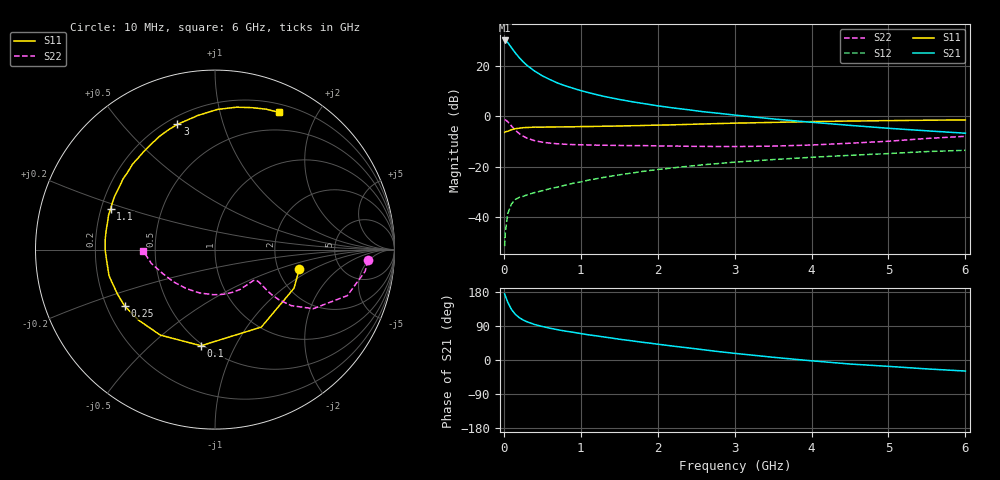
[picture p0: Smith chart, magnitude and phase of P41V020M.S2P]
! SIEMENS Small Signal Semiconductors
! BFP182
! Si NPN RF Bipolar Junction Transistor in SOT143
! VCE = 1 V  IC = 20 mA
! Common Emitter S-Parameters:  March  1996
# GHz  S  MA  R  50
!  f  S11  S21  S12  S22
! GHz  MAG  ANG  MAG  ANG  MAG  ANG  MAG  ANG
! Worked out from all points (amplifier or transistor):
!   36 points, 10 MHz to 6 GHz, reference 50 ohm
!   highest |S21| = 29.9 dB at 10 MHz (marker M1)
!   |S21| within 3 dB of that: start of sweep to 102.9 MHz
!   unconditionally stable (mu >= 1): start of sweep to 13.33 MHz; 343.8 MHz to end of sweep
!   at 250 MHz: K = 0.82, MSG = 26.6 dB, |S12| = -31.7 dB
!   at 1.4 GHz: K = 1.75, MAG = 10.4 dB, |S12| = -23.7 dB
!   at 6 GHz: K = 1.33, MAG = -0.1 dB, |S12| = -13.5 dB
!   S11 on the Smith chart (normalised r, x): 10 MHz: 2.63, -0.73; 100 MHz: 0.49, -0.74; 250 MHz: 0.27, -0.27; 1.1 GHz: 0.24, +0.18; 3 GHz: 0.24, +0.72; 6 GHz: 0.29, +1.53
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0.01  0.482 -12.8  31.39 174.3  0.0027 79.0  0.8538 -4.0
0.02  0.49 -26.1  31.28 168.8  0.0051 75.0  0.8456 -8.2
0.05  0.5029 -59.1  28.63 152.8  0.0118 68.6  0.7802 -19.2
0.1  0.5413 -98.3  22.53 133.2  0.0185 52.5  0.6391 -31.0
0.15  0.5655 -122.6  17.74 120.3  0.0226 45.2  0.5276 -36.3
0.2  0.5796 -137.3  14.37 111.8  0.0249 42.4  0.453 -38.1
0.25  0.5934 -147.9  11.92 105.6  0.026 41.0  0.4041 -38.5
0.3  0.5974 -155.5  10.13 101.0  0.0278 41.7  0.3692 -38.1
0.4  0.608 -166.0  7.797 93.7  0.031 43.5  0.3279 -37.1
0.5  0.6067 -173.9  6.284 88.4  0.0336 44.3  0.3064 -36.5
0.6  0.612 180.0  5.295 83.8  0.037 46.2  0.2936 -36.5
0.7  0.6143 174.5  4.514 79.9  0.0398 48.3  0.2845 -36.9
0.9  0.6172 166.4  3.569 73.2  0.0473 50.4  0.2745 -38.9
1.1  0.6243 158.6  2.927 66.5  0.0546 51.3  0.2705 -42.1
1.5  0.6392 145.8  2.145 54.9  0.0693 51.2  0.2644 -49.9
1.8  0.6544 136.4  1.794 46.8  0.0809 50.4  0.2625 -56.9
2.2  0.6754 125.9  1.458 36.6  0.0954 47.7  0.2574 -67.4
3  0.7287 106.7  1.053 17.6  0.1234 40.8  0.2514 -92.1
3.5  0.754 97.1  0.883 7.2  0.139 36.1  0.2562 -109.5
4.5  0.8024 81.4  0.659 -10.6  0.1686 27.0  0.2924 -142.0
5.5  0.8326 70.0  0.514 -23.5  0.2001 17.9  0.3634 -167.9
6  0.8437 64.9  0.461 -29.2  0.2119 12.4  0.4003 -179.0
